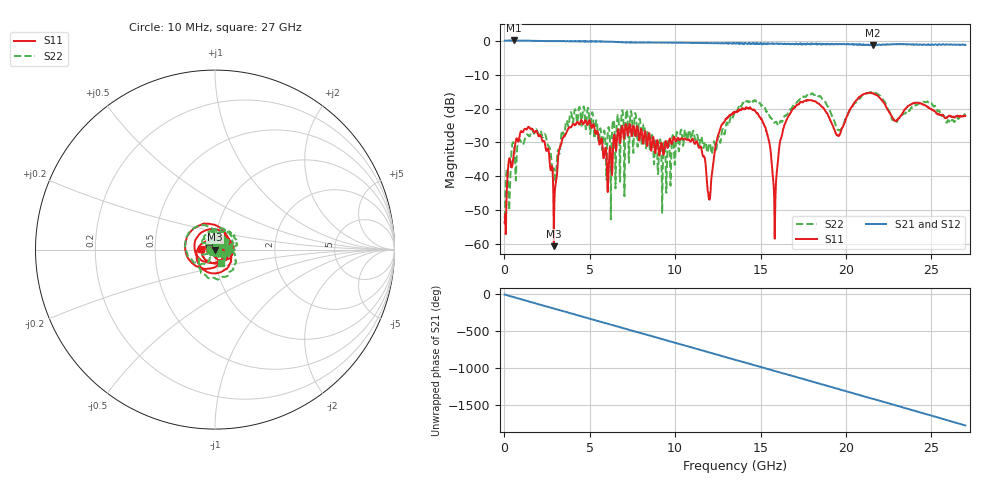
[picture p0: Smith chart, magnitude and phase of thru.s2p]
!Agilent Technologies,N5224A,MY51441447,A.10.00.00
!Agilent N5224A: A.10.00.00
!Date: Thursday, November 05, 2015 12:30:17
!Correction: S11(Full 2 Port(1,2))
!S21(Full 2 Port(1,2))
!S12(Full 2 Port(1,2))
!S22(Full 2 Port(1,2))
!S2P File: Measurements: S11, S21, S12, S22:
# Hz S  RI  R 50
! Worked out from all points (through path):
!   1601 points, 10 MHz to 27 GHz, reference 50 ohm
!   highest |S21| = 0.05 dB at 549.8 MHz (marker M1); lowest = -1.4 dB at 21.6 GHz (marker M2)
!   group delay of S21, straight-line fit = 182 ps
!   lowest |S11| = -60.6 dB at 2.895 GHz (marker M3), VSWR 1.00, Z = 50 - j0.0937 ohm
!   |S11| at or under -10 dB: start of sweep to end of sweep
!   |S22| runs from -52.7 to -15.2 dB; largest |S21 - S12| = 0.038
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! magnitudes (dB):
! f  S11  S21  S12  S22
! 10 MHz  -53.5  0.0  0.0  -52.3
! 263 MHz  -35.1  0.0  0.0  -49.7
! 549.8 MHz  -33.5  0.1  0.0  -30.7
! 1.967 GHz  -27.8  -0.1  -0.1  -27.5
! 2.895 GHz  -60.6  -0.1  -0.1  -37.6
! 3.384 GHz  -29.1  -0.2  -0.1  -26.5
! 4.514 GHz  -23.5  -0.2  -0.2  -25.1
! 6.15 GHz  -32.9  -0.3  -0.3  -26.9
! 7.213 GHz  -27.8  -0.6  -0.5  -22.5
! 9.018 GHz  -31.5  -0.6  -0.6  -36.7
! 11.16 GHz  -30.4  -0.7  -0.7  -29.0
! 11.99 GHz  -46.2  -0.8  -0.7  -30.3
! 12.61 GHz  -26.3  -0.7  -0.8  -29.6
! 13.51 GHz  -21.0  -0.8  -0.9  -20.7
! 15.14 GHz  -24.2  -1.1  -0.8  -19.3
! 15.83 GHz  -58.3  -0.9  -0.9  -24.1
! 16.51 GHz  -23.6  -1.0  -1.0  -22.0
! 18.01 GHz  -17.5  -0.8  -0.9  -15.5
! 19.54 GHz  -28.0  -1.1  -1.0  -26.3
! 21.6 GHz  -15.5  -1.4  -1.3  -15.2
! 22.51 GHz  -20.8  -1.1  -1.1  -20.5
! 27 GHz  -22.1  -1.2  -1.3  -21.7
